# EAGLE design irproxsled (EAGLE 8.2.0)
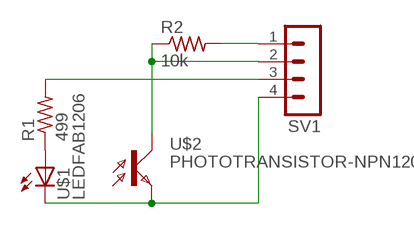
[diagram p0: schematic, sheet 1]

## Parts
R1  499  RES-US1206FAB  [R1206FAB]
R2  10k  RES-US1206FAB  [R1206FAB]
SV1  MA04-1  [MA04-1]
U$1  LEDFAB1206  [LED1206FAB]
U$2  PHOTOTRANSISTOR-NPN1206  [OP1206]

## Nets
N$1: R1.1 U$1.1(A)
N$2: SV1.4 U$1.2(C) U$2.EMITTER(E)
N$3: R2.2 SV1.1
N$4: R2.1 SV1.2 U$2.COLLECTOR(C)
N$10: R1.2 SV1.3

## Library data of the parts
R1 R2 = fab:RES-US: Resistor (US Symbol)
SV1 = con-lstb:MA04-1: PIN HEADER; OC_FARNELL: unknown; OC_NEWARK: unknown
U$1 = fab:LED: LED
U$2 = fab:PHOTOTRANSISTOR-NPN

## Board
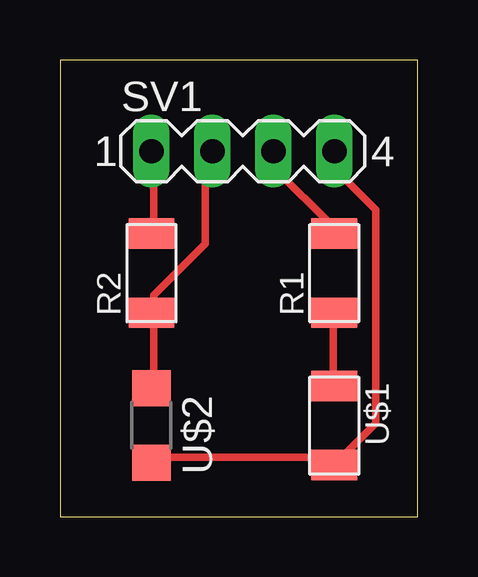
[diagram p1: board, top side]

Size 14.91 x 19.04 mm. Coordinates in mm from the lower left corner, seen from the top.
Outline: 0,0 14.91,0 14.91,19.04 0,19.04 0,0
Copper layers (1*16): Top 0.035mm / dielectric 1.5mm / Bottom 0.035mm
Design rules "default *": minimum track width 12mil, minimum drill 0.35mm, track to track 16mil, track to pad 16mil, pad to pad 16mil, via to via 16mil, smd to smd 16mil, copper to edge 40mil, drill to drill 6mil, minimum pad ring 10mil, minimum via ring 8mil, stop-mask expansion 4mil, vias tented up to drill 0mil, thermal gap 10mil

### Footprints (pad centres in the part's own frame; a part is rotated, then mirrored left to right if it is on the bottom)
R1206FAB = smd 1.27 x 1.905: 1 -1.651,0; 2 1.651,0
MA04-1 = drill 1.016 long: 1 -3.81,0; 2 -1.27,0; 3 1.27,0; 4 3.81,0
LED1206FAB = smd 1.27 x 1.905: 1 -1.651,0; 2 1.651,0
OP1206 = smd 1.5 x 1.6: COLLECTOR -1.55,0; EMITTER 1.55,0

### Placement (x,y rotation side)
R1  11.43,10.16 90 top
R2  3.81,10.16 90 top
SV1  7.62,15.24 0 top
U$1  11.43,3.81 270 top
U$2  3.81,3.81 270 top

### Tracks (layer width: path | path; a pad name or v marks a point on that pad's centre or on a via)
N$1
  Top 0.305: U$1.1 11.38,5.69 11.38,8.18 R1.1
N$2
  Top 0.305: U$2.EMITTER 3.91,2.49 11.38,2.49 U$1.2 11.73,2.49 13.16,3.91 13.16,12.8 11.73,14.22 11.73,14.94 SV1.4
N$3
  Top 0.305: R2.2 3.91,12.09 3.91,14.94 SV1.1
N$4
  Top 0.305: U$2.COLLECTOR 3.91,5.69 3.91,8.18 R2.1 3.91,8.53 3.91,9.25 6.04,11.38 6.04,14.94 SV1.2
N$10
  Top 0.305: SV1.3 8.89,14.58 11.38,12.09 R1.2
